ORGANIZATION_BLOCK MAIN:OB1
TITLE=Inversione di Marcia per M.A.T.
//Simulatore: 01
//Versione: 1.0
//Data: 10/02/2002
//
//------------ Descrizione del Controllo -----------------
// Il Programma gestisce l'inversione di marcia di un M.A.T.
// compresa la protezione del motore e le segnalazioni mediante
// l'uso di istruzioni di assegnazione e  autoritenuta software.
// Il motore M1 viene inserito tramite il pulsante SB2 per il
// funzionamento in "Marcia Avanti" o SB3 per la "Marcia Indietro".
// L'arresto del motore avviene tramite il pulsante SB1 o
// direttamente per l'intervento del relè termico FR.
// Si rammenta che per motivi di sicurezza il relè termico FR
// dovrà sempre intervenire anche via hardware per la sicura
// diseccitazione dei contattori.
// Il motore non può essere commutato dall'uno all'altro stato
// di marcia senza prima passare per l'arresto.
// Oltre all'interblocco hardware per impedire l'eccitazione
// contemporanea dei due contattori (sempre indispensabile!) il
// programma ne effettua anche uno software (doppio) interrogando
// sia lo stato delle uscite che lo stato dei contatti ausiliari
// dei contattori KM1 e KM2.
//

BEGIN
NETWORK 1 //Gestione Marcia Avanti
//
LD Q0.1
AN I0.0
A I0.4
O I0.2
A I0.1
A I0.5
AN Q0.0
= Q0.1

NETWORK 2 //Gestione  Marcia indietro
//
LD Q0.0
AN I0.4
A I0.0
O I0.3
A I0.1
A I0.5
AN Q0.1
= Q0.0

NETWORK 3 //Segnalazione Arresto Motore
//
LDN Q0.0
AN Q0.1
= Q0.2

NETWORK 4 //Segnalazione Marcia Indietro
//
LD Q0.0
= Q0.3

NETWORK 5 //Segnalazione marcia  Avanti
//
LD Q0.1
= Q0.4

NETWORK 6 //Segnalazione Relè Termico scattato
//
LDN I0.5
= Q0.5

END_ORGANIZATION_BLOCK

